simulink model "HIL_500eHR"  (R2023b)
settings: Solver=VariableStepAuto  StartTime=0.0  StopTime=Time  RelTol=1e-3
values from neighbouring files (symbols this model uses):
  BEV_mot = load("20241002_EM_Polito_Maps.mat")    [Init_FWD_500eHR.m]
undefined symbols (not defined in the file or in its folder): battery350V, bevGear, flip, motorDrive, T_EM_max, T_EM_max_cont, vehicle
libraries: fl_lib x38, nesl_utility x25, sdl_lib x11, slpidlib x3, simulink x3, ee_lib x2
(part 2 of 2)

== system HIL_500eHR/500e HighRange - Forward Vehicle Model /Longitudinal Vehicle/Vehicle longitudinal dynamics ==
  Discrete PID Controller : slpidlib/PID Controller  Controller=PID  Form=Parallel  TimeDomain=Discrete-time  UseExternalTs=off  SampleTime=-1  IntegratorMethod=Forward Euler  FilterMethod=Forward Euler  ControllerParametersSource=internal  P=0  I=0  UseKiTs=off  D=1  N=10  UseFilter=on  TunerSelectOption=Transfer Function Based (PID Tuner App)  InitialConditionSource=internal  InitialConditionForIntegrator=0  InitialConditionForFilter=0  DifferentiatorICPrevScaledInput=0  ExternalReset=none  TrackingMode=off  Kt=1  LimitOutput=off  SatLimitsSource=internal  UpperSaturationLimit=inf  LowerSaturationLimit=-inf  LinearizeAsGain=off  AntiWindupMode=none  Kb=1  LimitIntegrator=off  UpperIntegratorSaturationLimit=inf  LowerIntegratorSaturationLimit=-inf  POutMin=[]  POutMax=[]  IOutMin=[]  IOutMax=[]  DOutMin=[]  DOutMax=[]  NOutMin=[]  NOutMax=[]  SumOutMin=[]  SumOutMax=[]  SaturationOutMin=[]  SaturationOutMax=[]  PParamMin=[]  PParamMax=[]  IParamMin=[]  IParamMax=[]  DParamMin=[]  DParamMax=[]  NParamMin=[]  NParamMax=[]  KbParamMin=[]  KbParamMax=[]  KtParamMin=[]  KtParamMax=[]  KbOutMin=[]  KbOutMax=[]  KtOutMin=[]  KtOutMax=[]  IntegratorOutMin=[]  IntegratorOutMax=[]  FilterOutMin=[]  FilterOutMax=[]  SumI1OutMin=[]  SumI1OutMax=[]  SumI2OutMin=[]  SumI2OutMax=[]  SumI3OutMin=[]  SumI3OutMax=[]  SumI4OutMin=[]  SumI4OutMax=[]  SumDOutMin=[]  SumDOutMax=[]  DifferentiatorOutMin=[]  DifferentiatorOutMax=[]  FilterDiffOutCoefMin=[]  FilterDiffOutCoefMax=[]  ReciprocalOutMin=[]  ReciprocalOutMax=[]  SumDenOutMin=[]  SumDenOutMax=[]  SumNumOutMin=[]  SumNumOutMax=[]  DivideOutMin=[]  DivideOutMax=[]  UdiffTsProdOutMin=[]  UdiffTsProdOutMax=[]  NTsProdOutMin=[]  NTsProdOutMax=[]  UintegralTsProdOutMin=[]  UintegralTsProdOutMax=[]  UngainTsProdOutMin=[]  UngainTsProdOutMax=[]  ClampingZeroOutDataTypeStr=Inherit: Inherit via back propagation  ClampingZeroOutMin=[]  ClampingZeroOutMax=[]  FilterDenConstantOutDataTypeStr=Inherit: Inherit via back propagation  FilterDenConstantOutMin=[]  FilterDenConstantOutMax=[]  PCopyOutDataTypeStr=Inherit: Inherit via back propagation  PCopyOutMin=[]  PCopyOutMax=[]  NCopyOutDataTypeStr=Inherit: Inherit via back propagation  NCopyOutMin=[]  NCopyOutMax=[]  IntegratorContinuousStateAttributes=''  IntegratorStateMustResolveToSignalObject=off  IntegratorRTWStateStorageClass=Auto  FilterContinuousStateAttributes=''  FilterStateMustResolveToSignalObject=off  FilterRTWStateStorageClass=Auto  ParallelPVariant=InternalParameters  IdealPVariant=Disabled  IVariant=InternalParameters  DVariant=InternalParameters  IntegratorVariant=Discrete  SatVariant=Disabled  AWVariant=Passthrough  PCopyVariant=Disabled  TRVariant=Disabled  FdbkBlocksVariant=Forward  IdealPFdbkVariant=Disabled  SatFdbkVariant=Disabled  DerivativeFilterVariant=ForwardEulerFilter  NVariant=InternalParameters  NCopyVariant=Disabled  FilterICVariant=InternalICsFilter  IntegratorICVariant=InternalICs  ExternalResetVariant=Disabled  TRSumVariant=Passthrough  SumFdbkVariant=Disabled  SumVariant=Sum_PID  TsampFilterVariant=InternalTs  TsampNgainVariant=Passthrough  TsampIntegralVariant=Disabled_SignalSpec  ExternalSaturationOutDataTypeStr=Inherit: Same as second input
  Discrete PID Controller1 : slpidlib/PID Controller  Controller=PID  Form=Parallel  TimeDomain=Discrete-time  UseExternalTs=off  SampleTime=-1  IntegratorMethod=Forward Euler  FilterMethod=Forward Euler  ControllerParametersSource=internal  P=0  I=0  UseKiTs=off  D=1  N=5  UseFilter=on  TunerSelectOption=Transfer Function Based (PID Tuner App)  InitialConditionSource=internal  InitialConditionForIntegrator=0  InitialConditionForFilter=0  DifferentiatorICPrevScaledInput=0  ExternalReset=none  TrackingMode=off  Kt=1  LimitOutput=off  SatLimitsSource=internal  UpperSaturationLimit=inf  LowerSaturationLimit=-inf  LinearizeAsGain=off  AntiWindupMode=none  Kb=1  LimitIntegrator=off  UpperIntegratorSaturationLimit=inf  LowerIntegratorSaturationLimit=-inf  POutMin=[]  POutMax=[]  IOutMin=[]  IOutMax=[]  DOutMin=[]  DOutMax=[]  NOutMin=[]  NOutMax=[]  SumOutMin=[]  SumOutMax=[]  SaturationOutMin=[]  SaturationOutMax=[]  PParamMin=[]  PParamMax=[]  IParamMin=[]  IParamMax=[]  DParamMin=[]  DParamMax=[]  NParamMin=[]  NParamMax=[]  KbParamMin=[]  KbParamMax=[]  KtParamMin=[]  KtParamMax=[]  KbOutMin=[]  KbOutMax=[]  KtOutMin=[]  KtOutMax=[]  IntegratorOutMin=[]  IntegratorOutMax=[]  FilterOutMin=[]  FilterOutMax=[]  SumI1OutMin=[]  SumI1OutMax=[]  SumI2OutMin=[]  SumI2OutMax=[]  SumI3OutMin=[]  SumI3OutMax=[]  SumI4OutMin=[]  SumI4OutMax=[]  SumDOutMin=[]  SumDOutMax=[]  DifferentiatorOutMin=[]  DifferentiatorOutMax=[]  FilterDiffOutCoefMin=[]  FilterDiffOutCoefMax=[]  ReciprocalOutMin=[]  ReciprocalOutMax=[]  SumDenOutMin=[]  SumDenOutMax=[]  SumNumOutMin=[]  SumNumOutMax=[]  DivideOutMin=[]  DivideOutMax=[]  UdiffTsProdOutMin=[]  UdiffTsProdOutMax=[]  NTsProdOutMin=[]  NTsProdOutMax=[]  UintegralTsProdOutMin=[]  UintegralTsProdOutMax=[]  UngainTsProdOutMin=[]  UngainTsProdOutMax=[]  ClampingZeroOutDataTypeStr=Inherit: Inherit via back propagation  ClampingZeroOutMin=[]  ClampingZeroOutMax=[]  FilterDenConstantOutDataTypeStr=Inherit: Inherit via back propagation  FilterDenConstantOutMin=[]  FilterDenConstantOutMax=[]  PCopyOutDataTypeStr=Inherit: Inherit via back propagation  PCopyOutMin=[]  PCopyOutMax=[]  NCopyOutDataTypeStr=Inherit: Inherit via back propagation  NCopyOutMin=[]  NCopyOutMax=[]  IntegratorContinuousStateAttributes=''  IntegratorStateMustResolveToSignalObject=off  IntegratorRTWStateStorageClass=Auto  FilterContinuousStateAttributes=''  FilterStateMustResolveToSignalObject=off  FilterRTWStateStorageClass=Auto  ParallelPVariant=InternalParameters  IdealPVariant=Disabled  IVariant=InternalParameters  DVariant=InternalParameters  IntegratorVariant=Discrete  SatVariant=Disabled  AWVariant=Passthrough  PCopyVariant=Disabled  TRVariant=Disabled  FdbkBlocksVariant=Forward  IdealPFdbkVariant=Disabled  SatFdbkVariant=Disabled  DerivativeFilterVariant=ForwardEulerFilter  NVariant=InternalParameters  NCopyVariant=Disabled  FilterICVariant=InternalICsFilter  IntegratorICVariant=InternalICs  ExternalResetVariant=Disabled  TRSumVariant=Passthrough  SumFdbkVariant=Disabled  SumVariant=Sum_PID  TsampFilterVariant=InternalTs  TsampNgainVariant=Passthrough  TsampIntegralVariant=Disabled_SignalSpec  ExternalSaturationOutDataTypeStr=Inherit: Same as second input
  PS-Simulink Converter3 : nesl_utility/PS-Simulink Converter  PhysicalDomain=network_engine_domain  SubClassName=ps_output  LeftPortType=input  RightPortType=output  PseudoPeriodic=off  Frequencies=[]  VectorFormat=1-D array  Unit=m/s  AffineConversion=off
  Road Incline : fl_lib/Physical Signals/Sources/PS Constant  constant=road_grade rad
  Terminator : Terminator
  Transfer Fcn5 : TransferFcn  Denominator=[1/(2*pi*20) 1]
  Vehicle Body : sdl_lib/Tires & Vehicles/Vehicle Body  mass=vehicle.mass kg  n_w=2  x_f=vehicle.aCG m  x_r=vehicle.bCG m  y_c=vehicle.hCG m  mass_var=simscape.enum.onoff.off  g=9.81 m/s^2  liftoff_warning=simscape.enum.onoff.off  area=vehicle.Af m^2  Cd=vehicle.Cd  rho=1.225 kg/m^3  model_pitch=simscape.enum.onoff.off  inertia=4000 kg*m^2  suspension_model=sdl.enum.linearTLU.linear  k_f=1e4 N/m  b_f=1e4 N/(m/s)  k_r=1e4 N/m  b_r=1e4 N/(m/s)  k_f_TLU=[-2000, -1000, 0, 1000, 2000] N  x_f_TLU=[-.4, -.2, 0, .2, .4] m  b_f_TLU=[-200, -100, 0, 100, 200] N  v_f_TLU=[-4, -2, 0, 2, 4] m/s  k_r_TLU=[-2000, -1000, 0, 1000, 2000] N  x_r_TLU=[-.4, -.2, 0, .2, .4] m  b_r_TLU=[-200, -100, 0, 100, 200] N  v_r_TLU=[-4, -2, 0, 2, 4] m/s  interp_method=simscape.enum.interpolation.linear  extrap_method=simscape.enum.extrapolation.linear  model_hardstop=simscape.enum.onoff.off  upper_bound_f=.25 m  lower_bound_f=-.25 m  stop_k_f=1e6 N/m  stop_b_f=150 N/(m/s)  upper_bound_r=.25 m  lower_bound_r=-.25 m  stop_k_r=1e6 N/m  stop_b_r=150 N/(m/s)  initial_pitch=0 rad  initial_pitch_rate=0 rad/s  v_specify=on  v_priority=High  v=0 m/s  v_nominal_specify=off  v_nominal_unit=m/s  v_nominal_value=1
  Wind Velocity : fl_lib/Physical Signals/Sources/PS Constant  constant=0 m/s
  H : PMIOPort  Side=Left
  NF : PMIOPort  Port=2  Side=Right
  NR : PMIOPort  Port=3  Side=Left
  V_act : Outport  Unit=m/s  VectorParamsAs1DForOutWhenUnconnected=off
  a_act : Outport  Port=2  VectorParamsAs1DForOutWhenUnconnected=off
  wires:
  PS-Simulink Converter3/1 -> Transfer Fcn5/1, V_act/1  "Vehicle Speed [m/s]"
  Transfer Fcn5/1 -> Discrete PID Controller/1, [V_act]
  Discrete PID Controller/1 -> Discrete PID Controller1/1, a_act/1  "Vehicle Accel [m/s2]"
  Discrete PID Controller1/1 -> Terminator/1  "Vehicle Jerk [m/s2]"
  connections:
  Vehicle Body/RConn2 -- NF/RConn1
  Wind Velocity/RConn1 -- Vehicle Body/LConn3
  Road Incline/RConn1 -- Vehicle Body/RConn3
  Vehicle Body/RConn1 -- NR/RConn1
  PS-Simulink Converter3/LConn1 -- Vehicle Body/LConn2
  Vehicle Body/LConn1 -- H/RConn1

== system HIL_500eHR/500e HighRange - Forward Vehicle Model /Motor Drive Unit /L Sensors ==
  Ideal Torque Sensor2 : fl_lib/Mechanical/Mechanical Sensors/Ideal Torque Sensor
  Mechanical Rotational Reference3 : fl_lib/Mechanical/Rotational Elements/Mechanical Rotational Reference
  Motion Sensor3 : fl_lib/Mechanical/Mechanical Sensors/Ideal Rotational Motion Sensor  reference=foundation.enum.MeasurementReference.difference  acceleration_port=false  velocity_port=true  position_port=true  wrap_angle=simscape.enum.onoff.off  offset=0 rad
  PS-Simulink Converter1 : nesl_utility/PS-Simulink Converter  PhysicalDomain=network_engine_domain  SubClassName=ps_output  LeftPortType=input  RightPortType=output  PseudoPeriodic=off  Frequencies=[]  VectorFormat=inherit  Unit=inherit  AffineConversion=off
  PS-Simulink Converter3 : nesl_utility/PS-Simulink Converter  PhysicalDomain=network_engine_domain  SubClassName=ps_output  LeftPortType=input  RightPortType=output  PseudoPeriodic=off  Frequencies=[]  VectorFormat=inherit  Unit=inherit  AffineConversion=off
  Terminator : Terminator
  Terminator1 : Terminator
  S1 : PMIOPort  Side=Left
  L : PMIOPort  Port=2  Side=Right
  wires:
  PS-Simulink Converter1/1 -> Terminator/1  "T_left_input"
  PS-Simulink Converter3/1 -> Terminator1/1  "wL"
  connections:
  Motion Sensor3/RConn2 -- PS-Simulink Converter3/LConn1
  Ideal Torque Sensor2/RConn1 -- Motion Sensor3/LConn1 -- L/RConn1
  Motion Sensor3/RConn1 -- Mechanical Rotational Reference3/LConn1
  Ideal Torque Sensor2/RConn2 -- PS-Simulink Converter1/LConn1
  S1/RConn1 -- Ideal Torque Sensor2/LConn1

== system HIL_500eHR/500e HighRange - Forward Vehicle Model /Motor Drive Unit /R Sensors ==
  Ideal Torque Sensor1 : fl_lib/Mechanical/Mechanical Sensors/Ideal Torque Sensor
  Mechanical Rotational Reference2 : fl_lib/Mechanical/Rotational Elements/Mechanical Rotational Reference
  Motion Sensor2 : fl_lib/Mechanical/Mechanical Sensors/Ideal Rotational Motion Sensor  reference=foundation.enum.MeasurementReference.difference  acceleration_port=false  velocity_port=true  position_port=true  wrap_angle=simscape.enum.onoff.off  offset=0 rad
  PS-Simulink Converter2 : nesl_utility/PS-Simulink Converter  PhysicalDomain=network_engine_domain  SubClassName=ps_output  LeftPortType=input  RightPortType=output  PseudoPeriodic=off  Frequencies=[]  VectorFormat=inherit  Unit=inherit  AffineConversion=off
  PS-Simulink Converter4 : nesl_utility/PS-Simulink Converter  PhysicalDomain=network_engine_domain  SubClassName=ps_output  LeftPortType=input  RightPortType=output  PseudoPeriodic=off  Frequencies=[]  VectorFormat=inherit  Unit=inherit  AffineConversion=off
  Terminator : Terminator
  Terminator1 : Terminator
  R : PMIOPort  Side=Right
  S2 : PMIOPort  Port=2  Side=Left
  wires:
  PS-Simulink Converter2/1 -> Terminator1/1  "TR"
  PS-Simulink Converter4/1 -> Terminator/1  "wR"
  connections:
  Motion Sensor2/LConn1 -- Ideal Torque Sensor1/RConn1 -- R/RConn1
  Motion Sensor2/RConn1 -- Mechanical Rotational Reference2/LConn1
  Motion Sensor2/RConn2 -- PS-Simulink Converter4/LConn1
  PS-Simulink Converter2/LConn1 -- Ideal Torque Sensor1/RConn2
  Ideal Torque Sensor1/LConn1 -- S2/RConn1

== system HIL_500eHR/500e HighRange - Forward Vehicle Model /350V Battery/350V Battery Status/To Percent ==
  In1 : Inport
  Unit Conversion : UnitConversion
  Out1 : Outport  Unit=%
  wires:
  Unit Conversion/1 -> Out1/1
  In1/1 -> Unit Conversion/1

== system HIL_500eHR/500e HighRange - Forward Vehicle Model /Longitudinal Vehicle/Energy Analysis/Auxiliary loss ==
  Constant : Constant  Value=250
  Integrator3 : Integrator
  kWh1 : Gain  Gain=1/3600/1000
  auxiliary en. loss : Outport
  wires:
  Constant/1 -> Integrator3/1  "Aux Power Loss [W]"
  kWh1/1 -> auxiliary en. loss/1  "Aux Energy Loss [kWh]"
  Integrator3/1 -> kWh1/1

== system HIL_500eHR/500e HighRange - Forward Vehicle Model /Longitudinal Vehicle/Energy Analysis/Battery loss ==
  Battery_I : Inport
  POWER LOSS BATTERY : Subsystem
  Battery en. losses : Outport
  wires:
  Battery_I/1 -> POWER LOSS BATTERY/1(Battery_I)
  POWER LOSS BATTERY/1(Battery en. losses) -> Battery en. losses/1

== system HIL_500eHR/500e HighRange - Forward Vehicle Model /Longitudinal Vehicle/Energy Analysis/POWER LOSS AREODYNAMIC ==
  note: AERODYNAMIC POWER LOSS
  note: variables
  v_act : Inport
  Constant : Constant  Value=3
  Density : Constant  Value=1.225
  Drag coeff : Constant  Value=vehicle.Cd
  Frontal Area : Constant  Value=vehicle.Af
  Gain : Gain  Gain=0.5
  Integrator3 : Integrator
  Power : Math  Operator=pow
  Product : Product  Inputs=4
  kWh1 : Gain  Gain=1/3600/1000
  aero en. losses : Outport
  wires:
  Product/1 -> Integrator3/1  "Aero Power Loss [W]"
  v_act/1 -> [v_act]
  Density/1 -> Product/2
  Drag coeff/1 -> Product/3
  Frontal Area/1 -> Product/4
  Gain/1 -> Product/1
  [v_act] -> Power/1
  Constant/1 -> Power/2
  Power/1 -> Gain/1
  kWh1/1 -> aero en. losses/1  "Aero Energy Loss [kWh]"
  Integrator3/1 -> kWh1/1

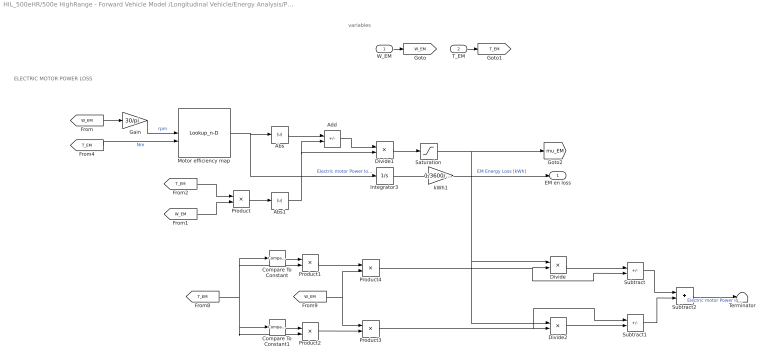
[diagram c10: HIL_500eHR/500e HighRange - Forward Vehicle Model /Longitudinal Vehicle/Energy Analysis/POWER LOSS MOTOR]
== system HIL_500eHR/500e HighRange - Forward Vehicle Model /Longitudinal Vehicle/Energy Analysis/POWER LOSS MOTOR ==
  note: ELECTRIC MOTOR POWER LOSS
  note: variables
  W_EM : Inport
  T_EM : Inport  Port=2
  Abs : Abs
  Abs1 : Abs
  Add : Sum  Inputs=-+
  Compare To Constant : simulink/Logic and Bit Operations/Compare To Constant  relop=>=  const=0  OutDataTypeStr=boolean
  Compare To Constant1 : simulink/Logic and Bit Operations/Compare To Constant  relop=<=  const=0  OutDataTypeStr=boolean
  Divide : Product  Inputs=/*
  Divide1 : Product  Inputs=*/
  Divide2 : Product  Inputs=/*
  Gain : Gain  Gain=30/pi
  Integrator3 : Integrator
  Motor efficiency map : Lookup_n-D  BreakpointsForDimension1=(BEV_mot.Speed(:,1))  BreakpointsForDimension2=flip(BEV_mot.Shaft_Torque(1,:))  Table=flip(BEV_mot.Total_Loss,2)  TableDataTypeStr=Inherit: Inherit from 'Table data'  InternalRulePriority=Speed  OutDataTypeStr=Inherit: Inherit via back propagation  RndMeth=Simplest
  Product{,1..4} (5 alike) : Product
  Saturation : Saturate  UpperLimit=1  LowerLimit=0
  Subtract : Sum  Inputs=+-
  Subtract1 : Sum  Inputs=+-
  Subtract2 : Sum
  Terminator : Terminator
  kWh1 : Gain  Gain=1/3600/1000
  EM en loss : Outport
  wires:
  W_EM/1 -> [W_EM]
  T_EM/1 -> [T_EM]
  Compare To Constant/1 -> Product1/1
  [T_EM] -> Product1/2, Compare To Constant/1, Product2/2, Compare To Constant1/1
  Product1/1 -> Product4/1
  Compare To Constant1/1 -> Product2/1
  Product2/1 -> Product3/2
  [W_EM] -> Product4/2, Product3/1
  Product4/1 -> Divide/2, Subtract/2
  Divide1/1 -> Saturation/1
  Product3/1 -> Divide2/2, Subtract1/1
  Divide/1 -> Subtract/1
  Divide2/1 -> Subtract1/2
  Motor efficiency map/1 -> Integrator3/1, Abs/1  "Electric motor Power loss [W]"
  Subtract/1 -> Subtract2/1
  Subtract1/1 -> Subtract2/2
  [W_EM] -> Product/2
  [T_EM] -> Product/1
  Product/1 -> Abs1/1
  Add/1 -> Divide1/1
  Saturation/1 -> [mu_EM], Divide2/1, Divide/1
  Abs/1 -> Add/1
  Abs1/1 -> Divide1/2, Add/2
  [W_EM] -> Gain/1
  Gain/1 -> Motor efficiency map/1  "rpm"
  [T_EM] -> Motor efficiency map/2  "Nm"
  kWh1/1 -> EM en loss/1  "EM Energy Loss [kWh]"
  Integrator3/1 -> kWh1/1
  Subtract2/1 -> Terminator/1  "Electric motor Power loss [W]"

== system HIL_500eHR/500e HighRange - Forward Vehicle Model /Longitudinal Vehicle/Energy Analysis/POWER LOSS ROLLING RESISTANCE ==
  note: ROLLING RESISTANCE LOSS
  V act : Inport
  Gain : Gain  Gain=9.81
  Integrator : Integrator
  Product : Product
  Product1 : Product
  Rolling coefficient : Constant  Value=vehicle.tireRRcoeff
  kWh2 : Gain  Gain=1/3600/1000
  mass vehicle : Constant  Value=vehicle.mass
  Out1 : Outport
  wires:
  Product/1 -> Product1/1
  mass vehicle/1 -> Gain/1
  Rolling coefficient/1 -> Product/2
  Gain/1 -> Product/1
  Product1/1 -> Integrator/1
  V act/1 -> Product1/2
  Integrator/1 -> kWh2/1
  kWh2/1 -> Out1/1  "Rolling Energy Loss [kWh]"

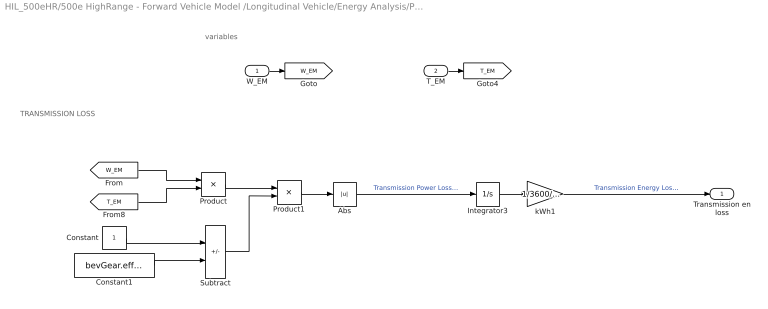
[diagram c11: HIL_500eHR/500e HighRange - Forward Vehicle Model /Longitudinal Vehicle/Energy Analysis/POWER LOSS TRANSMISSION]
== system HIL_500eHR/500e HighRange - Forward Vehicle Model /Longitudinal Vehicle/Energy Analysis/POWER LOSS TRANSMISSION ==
  note: TRANSMISSION LOSS
  note: variables
  W_EM : Inport
  T_EM : Inport  Port=2
  Abs : Abs
  Constant : Constant
  Constant1 : Constant  Value=bevGear.efficiency
  Integrator3 : Integrator
  Product : Product
  Product1 : Product
  Subtract : Sum  Inputs=+-
  kWh1 : Gain  Gain=1/3600/1000
  Transmission en loss : Outport
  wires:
  W_EM/1 -> [W_EM]
  T_EM/1 -> [T_EM]
  [W_EM] -> Product/1
  Abs/1 -> Integrator3/1  "Transmission Power Loss [W]"
  [T_EM] -> Product/2
  Constant/1 -> Subtract/1
  Constant1/1 -> Subtract/2
  Subtract/1 -> Product1/2
  Product/1 -> Product1/1
  Product1/1 -> Abs/1
  kWh1/1 -> Transmission en loss/1  "Transmission Energy Loss [kWh]"
  Integrator3/1 -> kWh1/1

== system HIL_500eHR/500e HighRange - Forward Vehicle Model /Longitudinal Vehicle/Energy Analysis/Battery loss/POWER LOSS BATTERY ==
  note: POWER BATTERY LOSS
  note: variables
  Battery_I : Inport
  Constant : Constant  Value=battery350V.internalResistance_Ohm  SampleTime=0.001
  Integrator3 : Integrator
  Product : Product
  Square : Math  Operator=square
  kWh1 : Gain  Gain=1/3600/1000
  Battery en. losses : Outport
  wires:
  Battery_I/1 -> [Battery_I]
  Product/1 -> Integrator3/1  "Battery Loss Power [W]"
  [Battery_I] -> Square/1
  Constant/1 -> Product/2
  Square/1 -> Product/1
  kWh1/1 -> Battery en. losses/1  "Battery Energy Loss [kWh]"
  Integrator3/1 -> kWh1/1

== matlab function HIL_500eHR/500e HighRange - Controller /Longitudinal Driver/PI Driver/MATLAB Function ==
function GasPedal = fcn(ReqTorque, Speed)

    % POLY23 GAS PEDAL MAP FROM MODEL RUNNING ON RDE SILVAGNI
    % Coefficients (with 95% confidence bounds):
    p00 =       4.342; % (4.128, 4.556)
    p10 =      0.9829; % (0.9533, 1.013)
    p01 =      0.5463; % (0.5147, 0.5778)
    p20 =    0.008702; % (0.007673, 0.009732)
    p11 =    -0.01185; % (-0.01455, -0.009155)
    p02 =  -0.0003168; % (-0.001127, 0.0004938)
    p21 =    0.001311; % (0.001249, 0.001374)
    p12 =  -0.0003258; % (-0.000355, -0.0002965)
    p03 =   7.114e-06; % (1.421e-06, 1.281e-05)

    GasPedal = p00 + p10*Speed + p01*ReqTorque + p20*Speed^2 + ...
               p11*Speed*ReqTorque + p02*ReqTorque^2 + p21*Speed^2*ReqTorque + ...
               p12*Speed*ReqTorque^2 + p03*ReqTorque^3;

    GasPedal = max(GasPedal,0);
